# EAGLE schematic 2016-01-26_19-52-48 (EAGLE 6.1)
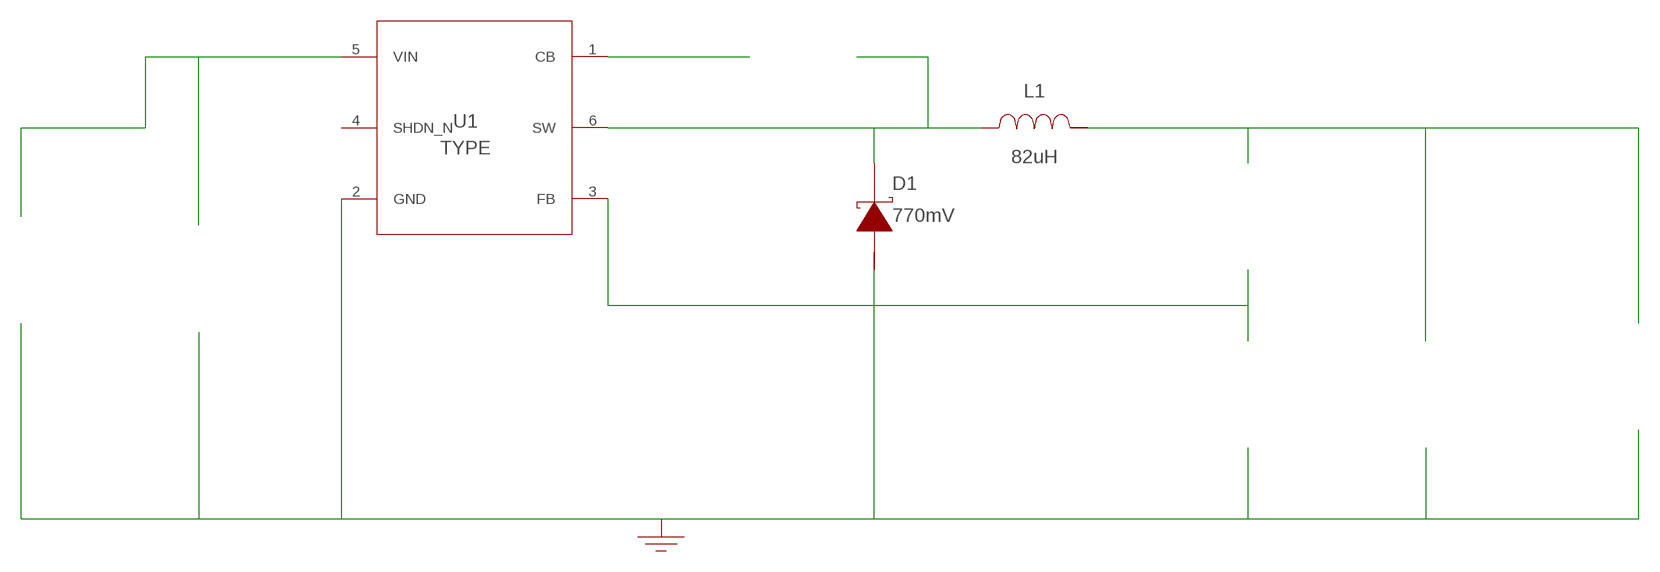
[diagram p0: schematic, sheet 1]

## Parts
CBOOT  100nF  GRM188R72A104KA35DGRM188R72A104KA35D  [0603]  (not placed on a sheet)
CIN  2.2uF  C3225X7R2A225K230ABC3225X7R2A225K230AB  [1210]  (not placed on a sheet)
COUT  4.7uF  GRM21BR61E475MA12LGRM21BR61E475MA12L  [0805]  (not placed on a sheet)
D1  770mV  DFLS1100-7DFLS1100-7  [PowerDI123]
GND  WB_GND  WB_GNDWB_GND  [WB_GND]
IOUT_1  WB_CURRENT_LOAD  WB_CURRENT_LOADWB_CURRENT_LOAD  [WB_CURRENT_LOAD]  (not placed on a sheet)
L1  82uH  ME3220-823KLBME3220-823KLB  [ME3220]
RFBB  6.04k  CRCW04026K04FKEDCRCW04026K04FKED  [0402]  (not placed on a sheet)
RFBT  88.7k  CRCW040288K7FKEDCRCW040288K7FKED  [0402]  (not placed on a sheet)
U1  LMR16006YDDCR  LMR16006YDDCRLMR16006YDDCR  [DDC0006A]
VIN  WB_BATTERY  WB_BATTERYWB_BATTERY  [WB_BATTERY]  (not placed on a sheet)

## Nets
0: Cin.2@2 Cout.2@2 D1.2(A) GND.1 Iout_1.-@2 Rfbb.2@2 U1.2(GND) Vin.-@2
1: Cin.1@1 U1.5(VIN) Vin.+@1
2: Rfbb.1@1 Rfbt.2@2 U1.3(FB)
3: Cboot.1@1 D1.1(K) L1.1 U1.6(SW)
4: Cout.1@1 Iout_1.+@1 L1.2 Rfbt.1@1
5: Cboot.2@2 U1.1(CB)
Unconnected: CBOOT.1 CBOOT.2 CIN.1 CIN.2 COUT.1 COUT.2 IOUT_1.1(+) IOUT_1.2(-) RFBB.1 RFBB.2 RFBT.1 RFBT.2 U1.4(SHDN_N) VIN.1(+) VIN.2(-)

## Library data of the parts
CBOOT = AcceleratedDesigns_Lib:GRM188R72A104KA35D; Cap: 1.0E-7; ESR: 0.0; IRMS: 0.0; Manufacturer_Name: MuRata; Manufacturer_Part_Number: GRM188R72A104KA35D; VDC: 100.0; Vendor: MuRata
CIN = AcceleratedDesigns_Lib:C3225X7R2A225K230AB; Cap: 2.2E-6; Datasheet_URL: http://product.tdk.com/capacitor/mlcc/en/documents/mlcc%5Fcommercial%5Fmidvoltage%5Fen.pdf; ESR: 0.0028; IRMS: 9.824718; Manufacturer_Name: TDK; Manufacturer_Part_Number: C3225X7R2A225K230AB; VDC: 100.0; Vendor: TDK
COUT = AcceleratedDesigns_Lib:GRM21BR61E475MA12L; Cap: 4.7E-6; Datasheet_URL: http://www.murata.com/products/catalog/pdf/c02e.pdf; ESR: 0.0020; IRMS: 7.29; Manufacturer_Name: MuRata; Manufacturer_Part_Number: GRM21BR61E475MA12L; VDC: 25.0; Vendor: MuRata
D1 = AcceleratedDesigns_Lib:DFLS1100-7; Datasheet_URL: http://www.diodes.com/datasheets/ds30497.pdf; Io: 1.0; Manufacturer_Name: Diodes Inc.; Manufacturer_Part_Number: DFLS1100-7; VFatIo: 0.77; VRRM: 100.0; Vendor: Diodes Inc.
GND = AcceleratedDesigns_Lib:WB_GND; Manufacturer_Name: WB_GND; Manufacturer_Part_Number: WB_GND; PowerPortType: POWER_GROUND; Value: Value
IOUT_1 = AcceleratedDesigns_Lib:WB_CURRENT_LOAD; Manufacturer_Name: WB_CURRENT_LOAD; Manufacturer_Part_Number: WB_CURRENT_LOAD; PowerPortType: POWER_GROUND; Value: Value
L1 = AcceleratedDesigns_Lib:ME3220-823KLB; DCR: 3.0; IDC: 0.34; L: 8.2E-5; Manufacturer_Name: Coilcraft; Manufacturer_Part_Number: ME3220-823KLB; Vendor: Coilcraft
RFBB = AcceleratedDesigns_Lib:CRCW04026K04FKED; Manufacturer_Name: Vishay-Dale; Manufacturer_Part_Number: CRCW04026K04FKED; Power: 0.063; Resistance: 6040.0; Tolerance: 1.0; Vendor: Vishay-Dale
RFBT = AcceleratedDesigns_Lib:CRCW040288K7FKED; Manufacturer_Name: Vishay-Dale; Manufacturer_Part_Number: CRCW040288K7FKED; Power: 0.063; Resistance: 88700.0; Tolerance: 1.0; Vendor: Vishay-Dale
U1 = AcceleratedDesigns_Lib:LMR16006YDDCR; CompType: IC; Manufacturer: Texas Instruments; Manufacturer_Name: Texas Instruments; Manufacturer_Part_Number: LMR16006YDDCR; MountType: SMT; PIN_COUNT: 6; PackageReference: DDC0006A; PartNumber: LMR16006YDDC; RefDes: RefDes; RoHS: Y; TYPE: TYPE; Value: Value
VIN = AcceleratedDesigns_Lib:WB_BATTERY; Manufacturer_Name: WB_BATTERY; Manufacturer_Part_Number: WB_BATTERY; PowerPortType: POWER_GROUND; Value: Value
